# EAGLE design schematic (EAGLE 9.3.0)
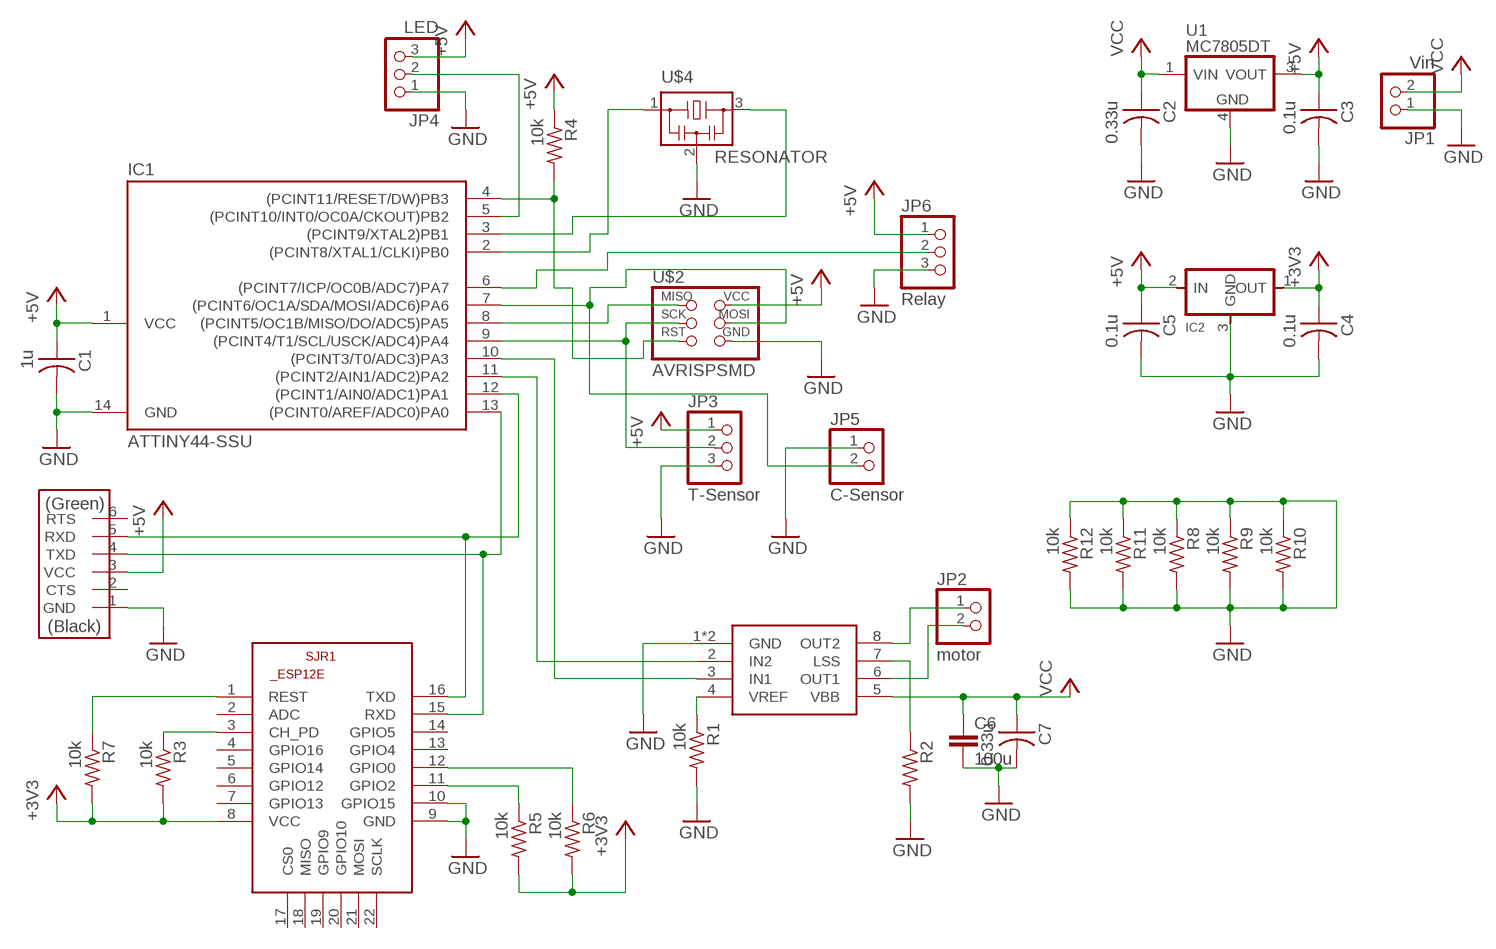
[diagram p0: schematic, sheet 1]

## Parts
C1  1u  CAP-US1206FAB  [C1206FAB]
C2  0.33u  CAP-US1206FAB  [C1206FAB]
C3  0.1u  CAP-US1206FAB  [C1206FAB]
C4  0.1u  CAP-US1206FAB  [C1206FAB]
C5  0.1u  CAP-US1206FAB  [C1206FAB]
C6  100u  C5/5  [C5B5]
C7  0.33u  CAP-US1206FAB  [C1206FAB]
IC1  ATTINY44-SSU  [SOIC14]
IC2  REGULATORSOT23  [SOT23]
JP1  Vin  PINHD-1X02_2.54-SMD-90°  [1X02SMD/90]
JP2  motor  PINHD-1X02_2.54-SMD-90°  [1X02SMD/90]
JP3  T-Sensor  PINHD-1X03_2.54-SMD-90°  [1X03SMD/90]
JP4  LED  PINHD-1X03_2.54-SMD-90°  [1X03SMD/90]
JP5  C-Sensor  PINHD-1X02_2.54-SMD-90°  [1X02SMD/90]
JP6  Relay  PINHD-1X03_2.54-SMD-90°  [1X03SMD/90]
R1  10k  RES-US1206FAB  [R1206FAB]
R2  RES-US1206FAB  [R1206FAB]
R3  10k  RES-US1206FAB  [R1206FAB]
R4  10k  RES-US1206FAB  [R1206FAB]
R5  10k  RES-US1206FAB  [R1206FAB]
R6  10k  RES-US1206FAB  [R1206FAB]
R7  10k  RES-US1206FAB  [R1206FAB]
R8  10k  RES-US1206FAB  [R1206FAB]
R9  10k  RES-US1206FAB  [R1206FAB]
R10  10k  RES-US1206FAB  [R1206FAB]
R11  10k  RES-US1206FAB  [R1206FAB]
R12  10k  RES-US1206FAB  [R1206FAB]
SJR1  ESP8266-12EESP12E  [ESP8266-ESP12E]
U1  MC7805DT  [DPAK-3]
U$1  FTDI-SMD-HEADER  [1X06SMD]
U$2  AVRISPSMD  [2X03SMD]
U$3  A4953-H-BRIDGE-MOTOR-DRIVER-PAD  [SOIC8_PAD]
U$4  RESONATOR  [EFOBM]

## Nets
+3V3: C4.1 IC2.1(OUT) R3.2 R5.2 R6.2 R7.2 SJR1.8(VCC)
+5V: C1.1 C3.1 C5.1 IC1.1(VCC) IC2.2(IN) JP3.1 JP4.3 JP6.1 R4.1 U1.3(VOUT) U$1.3(VCC) U$2.2(VCC)
GND: C1.2 C2.2 C3.2 C4.2 C5.2 C6.2 C7.2 IC1.14(GND) IC2.3(GND) JP1.1 JP3.3 JP4.1 JP5.1 JP6.3 R1.2 R2.2 R8.1 R8.2 R9.1 R9.2 R10.1 R10.2 R11.1 R11.2 R12.1 R12.2 SJR1.9(GND) SJR1.10(GPIO15) U1.4(GND) U$1.1(GND) U$2.6(GND) U$3.1(GND) U$3.GND U$4.2
N$1: IC1.4((PCINT11/RESET/DW)PB3) R4.2 U$2.5(RST)
N$2: IC1.2((PCINT8/XTAL1/CLKI)PB0) U$4.1
N$3: IC1.3((PCINT9/XTAL2)PB1) U$4.3
N$4: IC1.10((PCINT3/T0/ADC3)PA3) U$3.3(IN1)
N$5: IC1.11((PCINT2/AIN1/ADC2)PA2) U$3.2(IN2)
N$6: IC1.8((PCINT5/OC1B/MISO/DO/ADC5)PA5) U$2.1(MISO)
N$7: IC1.7((PCINT6/OC1A/SDA/MOSI/ADC6)PA6) JP5.2 U$2.4(MOSI)
N$8: R1.1 U$3.4(VREF)
N$10: R2.1 U$3.7(LSS)
N$11: IC1.12((PCINT1/AIN0/ADC1)PA1) SJR1.16(TXD) U$1.5(RXD)
N$12: JP2.1 U$3.8(OUT2)
N$13: IC1.13((PCINT0/AREF/ADC0)PA0) SJR1.15(RXD) U$1.4(TXD)
N$14: JP2.2 U$3.6(OUT1)
N$15: IC1.6((PCINT7/ICP/OC0B/ADC7)PA7) JP6.2
N$16: R6.1 SJR1.12(GPIO0)
N$17: IC1.5((PCINT10/INT0/OC0A/CKOUT)PB2) JP4.2
N$18: R3.1 SJR1.3(CH_PD)
N$19: R5.1 SJR1.11(GPIO2)
N$20: R7.1 SJR1.1(REST)
N$22: IC1.9((PCINT4/T1/SCL/USCK/ADC4)PA4) JP3.2 U$2.3(SCK)
VCC: C2.1 C6.1 C7.1 JP1.2 U1.1(VIN) U$3.5(VBB)
Unconnected: SJR1.2(ADC) SJR1.4(GPIO16) SJR1.5(GPIO14) SJR1.6(GPIO12) SJR1.7(GPIO13) SJR1.13(GPIO4) SJR1.14(GPIO5) SJR1.17(CS0) SJR1.18(MISO) SJR1.19(GPIO9) SJR1.20(GPIO10) SJR1.21(MOSI) SJR1.22(SCLK) U$1.2(CTS) U$1.6(RTS)

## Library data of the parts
C1-C5 C7 = eagle_fab:CAP-US
C6 = capacitor-wima:C: CAPACITOR
IC1 = eagle_fab:ATTINY44
IC2 = eagle_fab:REGULATOR
JP1 JP2 JP5 = pinhead-2:PINHD-1X02: PIN HEADER
JP3 JP4 JP6 = pinhead-2:PINHD-1X03: PIN HEADER
R1-R12 = eagle_fab:RES-US: Resistor (US Symbol)
SJR1 = esp12e:ESP8266-12E: ESP8266-12E Library for Eagle CAD The author not responsible for any damages or errors!. Created by Suhail jr.lt;/author>
U1 = _hhn_78xx_79xx_NCV78xx_d2pak_dpak:MC78*: 78xx SMD (D2PAK, DPAK) (MC)78xx..DT (DPAK-3; Rth,JA = 92 K/W) (MC)78xx..D2T (D2PAK-3; Rth,JA = 45 K/W @ 10x10mm copper area) Linear Voltage Regulators, Positive, 1 A (ON Semiconductor) Package dimenisions and soldering footprints acc. to ONSEMI specs. Source: http://onsemi.com Datasheet document#: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
U$1 = eagle_fab:FTDI-SMD-HEADER
U$2 = eagle_fab:AVRISP
U$3 = eagle_fab:A4953-H-BRIDGE-MOTOR-DRIVER-PAD
U$4 = eagle_fab:RESONATOR

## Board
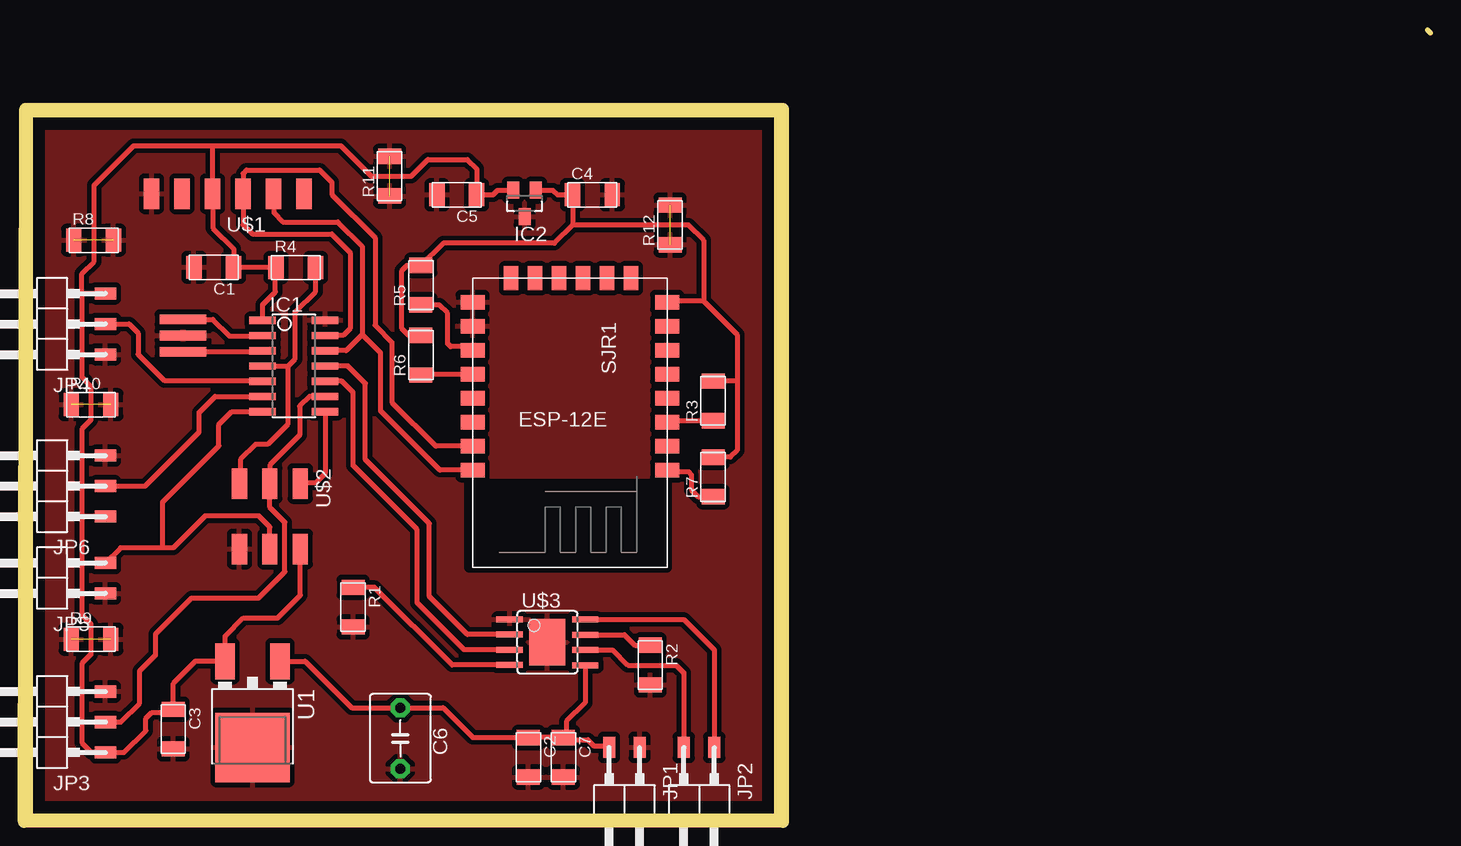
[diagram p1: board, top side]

Size 116.71 x 65.53 mm. Coordinates in mm from the lower left corner, seen from the top.
Outline: 116.71,65.28 116.46,65.53
Outline: 0,0 62.23,0 62.23,58.42 0,58.42 0,0
Copper layers (1*16): Top 0.035mm / dielectric 1.5mm / Bottom 0.035mm
Design rules "default *": minimum track width 16mil, minimum drill 0.35mm, track to track 16mil, track to pad 16mil, pad to pad 16mil, via to via 16mil, smd to smd 16mil, copper to edge 40mil, drill to drill 6mil, minimum pad ring 10mil, minimum via ring 8mil, stop-mask expansion 4mil, vias tented up to drill 0mil, thermal gap 16mil
Milling: 4 lines

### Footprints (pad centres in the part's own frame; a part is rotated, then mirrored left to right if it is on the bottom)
C1206FAB = smd 1.27 x 1.905: 1 -1.651,0; 2 1.651,0
C5B5 = drill 0.813 pad 1.6 octagon: 1 -2.54,0; 2 2.54,0
SOIC14 = smd 0.61 x 2.21: 1 -3.81,-2.603; 2 -2.54,-2.603; 3 -1.27,-2.603; 4 0,-2.603; 5 1.27,-2.603; 6 2.54,-2.603; 7 3.81,-2.603; 8 3.81,2.603; 9 2.54,2.603; 10 1.27,2.603; 11 0,2.603; 12 -1.27,2.603; 13 -2.54,2.603; 14 -3.81,2.603
SOT23 = smd 1 x 1.4: 1 -0.95,-1.1; 2 0.95,-1.1; 3 0,1.1
1X02SMD/90 = smd 1.016 x 1.778: 1 -1.27,-5.08; 2 1.27,-5.08
1X03SMD/90 = smd 1.016 x 1.778: 1 -1.27,-5.08; 2 1.27,-5.08; 3 3.81,-5.08
R1206FAB = smd 1.27 x 1.905: 1 -1.651,0; 2 1.651,0
ESP8266-ESP12E = smd 2 x 1.2: 1 -7.62,5.84; 2 -7.62,3.84; 3 -7.62,1.84; 4 -7.62,-0.16; 5 -7.62,-2.16; 6 -7.62,-4.16; 7 -7.62,-6.16; 8 -7.62,-8.16; 9 8.58,-8.16; 10 8.58,-6.16; 11 8.58,-4.16; 12 8.58,-2.16; 13 8.58,-0.16; 14 8.58,1.84; 15 8.58,3.84; 16 8.58,5.84 | smd 1.2 x 2: 17 -4.62,-10.16; 18 -2.62,-10.16; 19 -0.62,-10.16; 20 1.38,-10.16; 21 3.38,-10.16; 22 5.38,-10.16
DPAK-3 = smd 1.6 x 3: 1 -2.286,-7.18; 3 2.286,-7.18 | smd 6.2 x 5.8: 4 0,0
1X06SMD = smd 2.54 x 1.27: 1 0,6.35; 2 0,3.81; 3 0,1.27; 4 0,-1.27; 5 0,-3.81; 6 0,-6.35
2X03SMD = smd 2.54 x 1.27: 1 -2.54,2.54; 2 2.92,2.54; 3 -2.54,0; 4 2.92,0; 5 -2.54,-2.54; 6 2.92,-2.54
SOIC8_PAD = smd 0.5 x 2.2: 1 -1.905,-3.154; 2 -0.645,-3.154; 3 0.625,-3.154; 4 1.895,-3.154; 5 1.905,3.154; 6 0.635,3.154; 7 -0.635,3.154; 8 -1.905,3.154 | smd 3.886 x 2.997: GND 0,0
EFOBM = smd 0.8 x 3.9: 1 -1.35,0; 2 0,0; 3 1.35,0

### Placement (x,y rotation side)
C1  15.32,45.75 180 top
C2  41.53,4.89 270 top
C3  11.94,7.24 270 top
C4  46.86,51.8 0 top
C5  35.56,51.8 180 top
C6  30.86,6.48 270 top
C7  44.45,4.89 270 top
IC1  22,37.52 270 top
IC2  41.21,51.07 180 top
JP1  49.53,0.64 180 top
JP2  55.75,0.64 180 top
JP3  1.21,6.56 90 top
JP4  1.21,39.75 90 top
JP5  1.21,19.83 90 top
JP6  1.21,26.23 90 top
R1  26.92,17.41 270 top
R2  51.69,12.58 270 top
R3  56.93,34.61 90 top
R4  22.15,45.72 0 top
R5  32.58,44.26 90 top
R6  32.58,38.42 90 top
R7  56.93,28.26 90 top
R8  5.3,48.01 0 top
R9  5.08,14.73 0 top
R10  5.08,34.29 0 top
R11  29.97,53.34 90 top
R12  53.34,49.28 90 top
SJR1  45.47,34.67 180 top
U1  18.54,5.71 180 top
U$1  16.48,51.87 90 top
U$2  19.99,25.17 270 top
U$3  43.12,14.48 270 top
U$4  12.75,40.06 270 top

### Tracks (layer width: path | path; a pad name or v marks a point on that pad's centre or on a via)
+3V3
  Top 0.406: IC2.1 43.58,52.17 43.96,51.8 C4.1 45.21,49.28 | 56.13,42.93 56.13,48.01 54.86,49.28 45.21,49.28 | SJR1.8 53.09,42.93 56.13,42.93 | R6.2 31.56,40.07 30.99,40.64 30.99,45.47 31.43,45.91 R5.2 34.42,47.75 43.69,47.75 45.21,49.28 | 58.93,36.32 58.93,40.13 56.13,42.93 | 58.93,36.32 58.93,30.48 58.36,29.91 R7.2 | R3.2 56.99,36.32 58.93,36.32
+5V
  Top 0.406: 20.47,45.74 C1.1 16.97,47.3 15.24,49.02 15.24,51.84 U$1.3 15.24,51.89 15.24,55.88 | 20.47,45.74 R4.1 | U$2.2 22.53,18.41 20.63,16.51 17.78,16.51 16.26,14.99 U1.3 13.78,12.89 11.94,11.05 C3.1 11.68,8.64 10.16,8.64 9.65,8.13 9.65,7.11 7.83,5.29 JP3.1 5.12,5.29 4.32,6.1 4.32,12.7 5.08,13.46 5.08,16 4.32,16.76 4.32,24.96 | IC1.1 19.39,42.63 20.45,43.69 20.45,45.72 20.47,45.74 | IC2.2 38.97,52.17 38.59,51.8 C5.1 37.21,53.98 36.45,54.74 33.15,54.74 31.75,53.34 28.45,53.34 25.91,55.88 15.24,55.88 | 4.32,43.56 JP4.3 4.51,43.56 | 4.32,24.96 4.32,32.26 5.08,33.02 5.08,35.81 4.32,36.58 4.32,43.56 | JP6.1 4.32,24.96 | 4.32,43.56 4.32,45.21 5.33,46.23 5.33,52.58 8.64,55.88 15.24,55.88
GND  (5 unrouted)
  pour Top (isolate 0.406): -3.17,-3.05 65.81,-3.05 65.81,61.93 -3.17,61.93
N$1
  Top 0.406: R4.2 23.8,43.74 22.1,42.04 22.1,38.1 21.46,37.47 | IC1.4 19.44,37.47 21.46,37.47 | 21.46,37.47 21.46,32.64 19.81,30.99 18.8,30.99 17.53,29.72 17.53,27.79 U$2.5
N$2
  Top 0.406: U$4.1 15.24,41.41 16.64,40.01 19.34,40.01 IC1.2
N$3
  Top 0.406: 12.91,38.86 U$4.3 19.31,38.71 IC1.3 19.32,38.86
N$4
  Top 0.406: U$3.3 36.19,13.85 32.26,17.78 32.26,23.88 26.92,29.21 26.92,35.31 25.98,36.25 IC1.10
N$5
  Top 0.406: IC1.11 26.49,37.52 27.94,36.07 27.94,29.72 33.27,24.38 33.27,18.29 36.44,15.12 U$3.2
N$6
  Top 0.406: U$2.1 22.48,27.76 23.82,27.76 24.6,28.54 IC1.8
N$7
  Top 0.406: U$2.4 19.99,24.08 19.05,25.02 14.61,25.02 11.94,22.35 11.05,22.35 | 11.05,22.35 11.05,26.16 15.75,30.86 15.75,32.64 16.82,33.71 IC1.7 | 11.05,22.35 7.54,22.35 JP5.2
N$8
  Top 0.406: U$3.4 35.17,12.58 28.69,19.06 R1.1
N$10
  Top 0.406: U$3.7 49.53,15.11 50.41,14.23 R2.1
N$11
  Top 0.406: U$1.5 20.32,51.84 20.32,50.29 21.08,49.53 25.65,49.53 27.69,47.5 27.69,40.13 | IC1.12 26.34,38.79 27.69,40.13 | SJR1.16 34.16,28.83 29.21,33.78 29.21,38.61 27.69,40.13
N$12
  Top 0.406: U$3.8 54.48,16.38 57.02,13.84 JP2.1
N$13
  Top 0.406: IC1.13 26.09,40.06 26.67,40.64 26.67,46.99 25.15,48.51 18.54,48.51 17.75,49.3 U$1.4 17.75,53.57 18.03,53.85 24.13,53.85 25.15,52.83 25.15,51.82 28.75,48.21 28.75,40.89 30.17,39.48 30.17,34.48 33.82,30.83 SJR1.15
N$14
  Top 0.406: U$3.6 48.56,13.84 49.83,12.57 53.85,12.57 54.48,11.94 JP2.2
N$15
  Top 0.406: JP6.2 9.6,27.5 14.1,32 14.1,33.66 15.42,34.98 IC1.6
N$16
  Top 0.406: R6.1 32.64,36.83 SJR1.12
N$17
  Top 0.406: JP4.2 8.26,41.02 9.02,40.26 9.02,38.48 11.18,36.32 19.21,36.32 19.34,36.2 IC1.5
N$18
  Top 0.406: SJR1.3 53.21,32.96 R3.1
N$19
  Top 0.406: SJR1.11 36.6,39.12 35.05,39.12 34.8,39.37 34.8,41.91 34.1,42.61 R5.1
N$20
  Top 0.406: SJR1.1 53.22,28.7 54.86,28.7 55.12,28.45 55.12,27.18 55.69,26.61 R7.1
N$22
  Top 0.406: IC1.9 23.29,34.98 22.48,34.16 22.48,31.75 19.99,29.26 U$2.3 19.99,25.73 21.23,24.49 21.23,20.34 19.05,18.16 13.46,18.16 10.48,15.18 10.48,13.42 9.14,12.09 9.14,9.4 7.58,7.83 JP3.2
VCC
  Top 0.406: U1.1 22.92,12.89 26.8,9.02 C6.1 34.42,9.02 36.89,6.54 C2.1 C7.1 | JP1.2 48.13,5.84 46.99,5.84 46.48,6.35 44.64,6.35 C7.1 | U$3.5 46.27,9.44 44.7,7.87 44.7,6.79 C7.1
